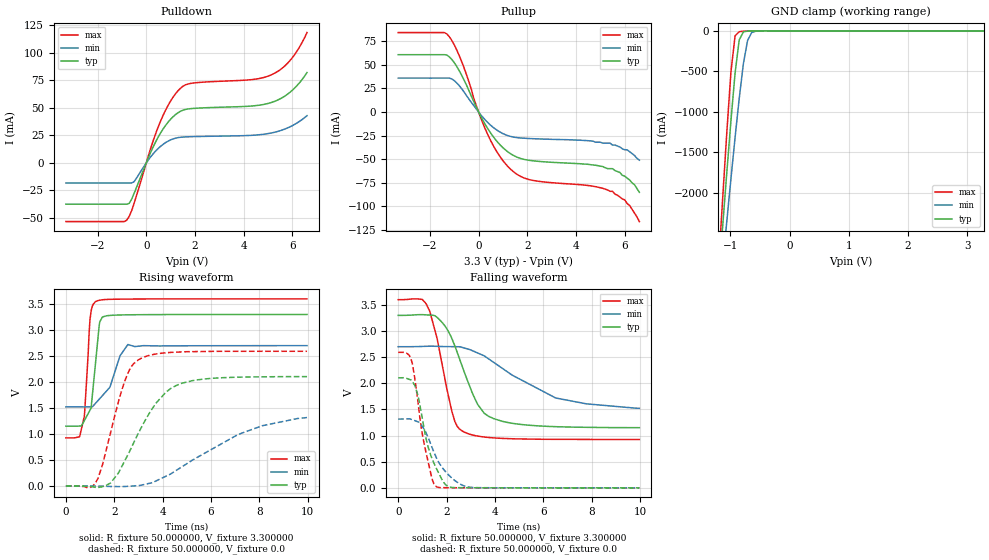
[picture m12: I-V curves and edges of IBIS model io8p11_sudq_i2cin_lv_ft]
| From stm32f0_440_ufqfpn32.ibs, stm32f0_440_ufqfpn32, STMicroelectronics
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|   Model io8p11_sudq_i2cin_lv_ft
[Model]  io8p11_sudq_i2cin_lv_ft
Model_type I/O
Polarity   Non-Inverting
Enable   Active-Low
Vinl =   0.990000V
Vinh =   2.310000V
Vmeas =  1.650000V
Cref =   30.000000pF
Rref =   100.000000M
Vref =   0.0V
C_comp   2.070000pF   1.996000pF   2.160200pF
[Temperature Range]   25.000000   0.125000k   -40.000000
[Pullup Reference]   3.300000V   2.700000V   3.600000V
[Pulldown Reference]   0.0V   0.0V   0.0V
[POWER Clamp Reference]   3.300000V   2.700000V   3.600000V
[GND Clamp Reference]   0.0V   0.0V   0.0V
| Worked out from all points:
|   slope of the pulldown table from 0 to 0.495 V, typ, clamps not added: 20.9 ohm
|   slope of the pullup table from 0 to 0.495 V, typ, clamps not added: 22.2 ohm
|   GND clamp passes 1 mA (typ) near -0.64 V on its own axis
|   rising waveform, R_fixture 50.000000, V_fixture 3.300000: 20-80 % time 272ps typ, 664ps min, 195ps max; typ from 1.15 V to 3.3 V
|   rising waveform, R_fixture 50.000000, V_fixture 0.0: 20-80 % time 1.54ns typ, 3.05ns min, 906ps max; typ from 0 V to 2.1 V
|   falling waveform, R_fixture 50.000000, V_fixture 3.300000: 20-80 % time 1.11ns typ, 2.61ns min, 732ps max; typ from 3.3 V to 1.15 V
|   falling waveform, R_fixture 50.000000, V_fixture 0.0: 20-80 % time 673ps typ, 896ps min, 537ps max; typ from 2.1 V to 0 V
[Pulldown]
|Voltage   I(typ)   I(min)   I(max)
-3.3V     -37.45mA   -18.2mA    -53.24mA
-800mV    -37.45mA   -18.2mA    -51.9mA
-700mV    -36.7mA    -18.2mA    -48.48mA
-500mV    -27.71mA   -17.01mA   -36.66mA
200mV     10.57mA    6.084mA    14.57mA
500mV     23.91mA    13.38mA    33.24mA
900mV     37.17mA    19.87mA    52.48mA
1.3V      45.55mA    23.01mA    65.5mA
1.8V      49.29mA    23.83mA    72.18mA
5.1V      54.68mA    27.07mA    79.72mA
5.9V      64.2mA     32.82mA    93.01mA
6.6V      82.13mA    42.97mA    118.4mA
[Pullup]
|Voltage   I(typ)   I(min)   I(max)
-3.3V     60.68mA    35.91mA    84.08mA
-1.4V     60.68mA    35.91mA    84.08mA
-1.2V     58.37mA    35.91mA    79.67mA
-700mV    39.18mA    24.86mA    53.7mA
0V        90fA       16.1pA     0A
400mV     -18.61mA   -11.78mA   -25.23mA
900mV     -35.28mA   -21.55mA   -48mA
1.5V      -46.91mA   -26.86mA   -64.57mA
2.2V      -51.57mA   -28.22mA   -72.25mA
5.5V      -60mA      -35mA      -84mA
6V        -68mA      -40mA      -93mA
6.6V      -85mA      -51mA      -116mA
[GND_clamp]
|Voltage   I(typ)   I(min)   I(max)
-3.3V     -9.366A    -9.678A    -9.859A
-1.2V     -3.091A    -3.431A    -2.911A
-1.13V    -2.415A    -2.888A    -2.072A
-1.06V    -1.751A    -2.352A    -1.259A
-990mV    -1.112A    -1.826A    -509.3mA
-920mV    -522.9mA   -1.315A    -61.61mA
-850mV    -112.5mA   -833.8mA   -10.22mA
-780mV    -13.59mA   -408.1mA   -5.256mA
-710mV    -3.081mA   -122.1mA   -2.635mA
-640mV    -945.2uA   -21.36mA   -905.7uA
-570mV    -199.6uA   -4.142mA   -156.8uA
3.28V     0A         0A         0A
[POWER_clamp]
|Voltage   I(typ)   I(min)   I(max)
-3.28V    0A         0A         0A
0V        0A         0A         0A
[Ramp]
| variable   typ   min   max
dV/dt_r  1.26186/1.53560n   0.74040/3.03782n   1.55460/0.90540n
dV/dt_f  1.28832/1.10495n   0.68772/2.59684n   1.60471/0.73153n
R_load = 50.000000
[Rising Waveform]
R_fixture= 50.000000
V_fixture= 3.300000
V_fixture_min= 2.700000
V_fixture_max= 3.600000
|time   V(typ)   V(min)   V(max)
0s        1.151V     1.522V     925.5mV
560.6ps   1.153V     1.522V     946mV
760.8ps   1.255V     1.521V     1.334V
1.001ns   1.462V     1.522V     3.216V
1.221ns   2.345V     1.588V     3.545V
1.381ns   3.106V     1.671V     3.572V
1.502ns   3.245V     1.734V     3.582V
1.822ns   3.281V     1.903V     3.591V
2.563ns   3.293V     2.721V     3.596V
9.97ns    3.3V       2.7V       3.6V
[Rising Waveform]
R_fixture= 50.000000
V_fixture= 0.0
V_fixture_min= 0.0
V_fixture_max= 0.0
|time   V(typ)   V(min)   V(max)
0s        -16.78uV   -27.94uV   -14.15uV
1.201ns   -24.19mV   -1.024mV   41.72mV
1.502ns   -14.8mV    -4.282mV   391mV
1.842ns   55.49mV    -9.454mV   1.014V
2.382ns   437.4mV    -11.31mV   1.945V
3.003ns   1.02V      8.087mV    2.429V
3.744ns   1.602V     100.8mV    2.541V
4.805ns   1.978V     371.1mV    2.579V
7.127ns   2.093V     991.5mV    2.591V
9.97ns    2.104V     1.316V     2.591V
[Falling Waveform]
R_fixture= 50.000000
V_fixture= 3.300000
V_fixture_min= 2.700000
V_fixture_max= 3.600000
|time   V(typ)   V(min)   V(max)
0s        3.3V       2.7V       3.6V
1.001ns   3.314V     2.706V     3.602V
1.301ns   3.304V     2.71V      3.383V
1.602ns   3.262V     2.707V     2.87V
2.222ns   2.851V     2.701V     1.456V
2.663ns   2.303V     2.684V     1.084V
3.283ns   1.597V     2.581V     990.8mV
3.964ns   1.322V     2.395V     955.2mV
6.507ns   1.171V     1.72V      928.3mV
9.97ns    1.151V     1.522V     925.5mV
[Falling Waveform]
R_fixture= 50.000000
V_fixture= 0.0
V_fixture_min= 0.0
V_fixture_max= 0.0
|time   V(typ)   V(min)   V(max)
0s        2.104V     1.316V     2.591V
360.4ps   2.092V     1.32V      2.573V
580.6ps   2.034V     1.304V     2.386V
800.8ps   1.788V     1.266V     1.711V
1.081ns   1.112V     1.118V     825.2mV
1.401ns   557mV      766.8mV    171.4mV
1.602ns   349.4mV    550.9mV    16.75mV
2.062ns   25.04mV    256.1mV    2.563mV
3.003ns   1.784mV    10mV       1.003mV
9.97ns    -16.78uV   -27.94uV   -14.15uV
